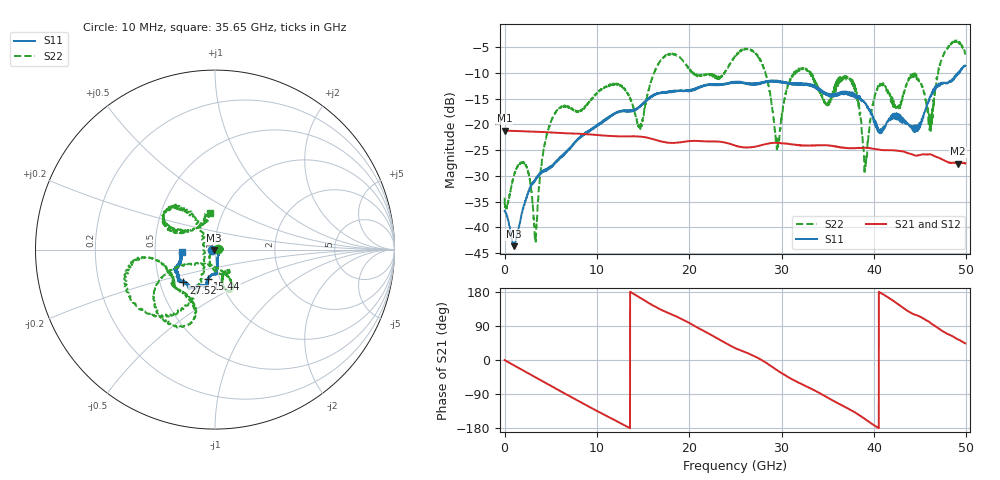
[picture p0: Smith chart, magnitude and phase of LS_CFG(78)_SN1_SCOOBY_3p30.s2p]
!Keysight Technologies,N5245B,MY58422026,A.13.80.08
!Date: Thursday, March 19, 2020 23:51:29
!Correction: S11(Full 2 Port(1,2))
!S21(Full 2 Port(1,2))
!S12(Full 2 Port(1,2))
!S22(Full 2 Port(1,2))
!S2P File: Measurements: S11, S21, S12, S22:
# Hz S DB R 50.0
!freq dBS11 angS11 dBS21 angS21 dBS12 angS12 dBS22 angS22
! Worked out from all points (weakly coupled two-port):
!   4991 points, 10 MHz to 49.91 GHz, reference 50 ohm
!   highest |S21| = -21.19 dB at 10 MHz (marker M1); lowest = -27.6 dB at 49.11 GHz (marker M2)
!   lowest |S11| = -43.7 dB at 990 MHz (marker M3), VSWR 1.01, Z = 49.5 - j0.436 ohm
!   |S11| at or under -10 dB: start of sweep to 49.12 GHz; 49.17411 GHz to 49.22027 GHz (46.17 MHz wide, 0.0938 % of centre)
!   |S22| runs from -42.8 to -3.7 dB; largest |S21 - S12| = 0.00084
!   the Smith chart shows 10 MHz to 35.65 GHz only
!   S11 on the Smith chart (normalised r, x): 10 MHz: 0.97, -0.01; 15.44 GHz: 0.87, -0.30; 27.52 GHz: 0.66, -0.26; 35.65 GHz: 0.69, -0.02
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1e7  -36.79 -168.9  -21.19 -0.3  -21.18 -0.3  -34.27 2.6
9.9e8  -43.68 -137.8  -21.26 -13.7  -21.26 -13.7  -30.06 -27.1
2.36e9  -34.23 -55.8  -21.35 -32.4  -21.34 -32.3  -28.09 19.3
3.34e9  -30.66 -56.7  -21.42 -45.6  -21.41 -45.5  -41.76 129.8
5.05e9  -28.29 -63.0  -21.56 -68.8  -21.56 -68.8  -19.28 -95.9
8.33e9  -22.42 -79.7  -21.84 -112.4  -21.83 -112.4  -17.22 -66.9
1.544e10  -15.35 -104.0  -22.58 153.0  -22.57 153.1  -14.70 -153.9
1.665e10  -14.00 -103.2  -23.14 136.4  -23.14 136.4  -8.25 -147.6
2.496e10  -11.86 -124.3  -24.06 31.8  -24.06 32.0  -6.83 -170.8
2.752e10  -11.89 -134.0  -24.17 4.3  -24.16 4.6  -6.85 -125.0
2.954e10  -11.67 -141.3  -23.58 -27.2  -23.58 -26.9  -24.05 -175.7
3.103e10  -11.98 -146.1  -23.86 -49.4  -23.88 -49.2  -10.76 127.9
3.328e10  -12.39 -156.3  -24.08 -76.9  -24.09 -76.5  -10.52 156.0
3.565e10  -14.59 -175.1  -24.19 -108.2  -24.13 -107.7  -13.75 97.1
3.78e10  -14.46 177.4  -24.63 -136.2  -24.57 -136.3  -11.92 135.1
3.905e10  -15.76 173.4  -24.54 -155.9  -24.53 -156.1  -28.72 -122.7
4.03e10  -20.13 159.3  -24.83 -176.5  -24.83 -176.7  -13.28 -6.4
4.16e10  -18.98 107.8  -25.01 164.4  -25.04 164.3  -14.02 25.3
4.445e10  -20.74 55.8  -26.05 119.5  -26.06 119.8  -10.29 -15.7
4.614e10  -14.47 8.5  -25.81 97.7  -25.83 97.8  -21.11 -46.2
4.911e10  -10.09 -12.9  -27.63 54.2  -27.64 54.3  -3.84 -44.3
4.991e10  -8.55 -13.3  -27.56 43.9  -27.59 43.9  -6.18 -28.9
